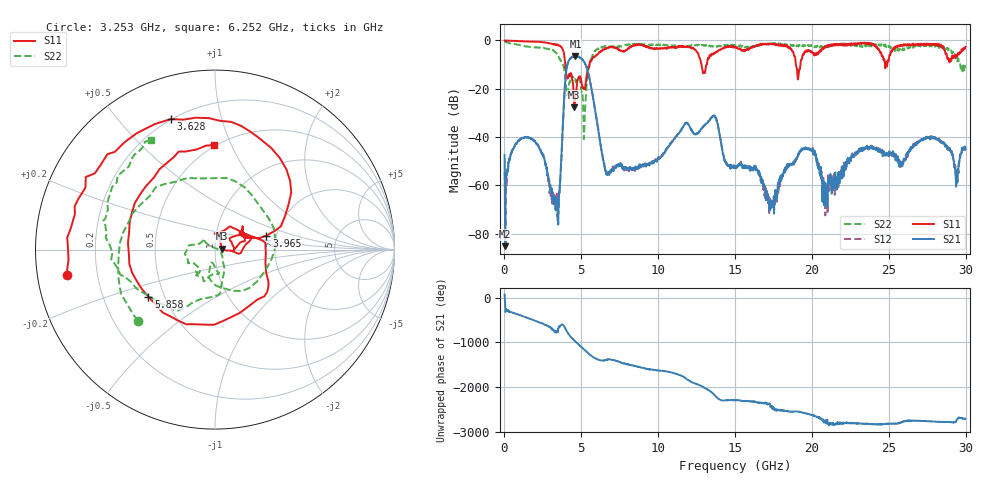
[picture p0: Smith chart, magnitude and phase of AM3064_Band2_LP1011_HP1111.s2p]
# Hz S DB R 50.0
!freq dBS11 angS11 dBS21 angS21 dBS12 angS12 dBS22 angS22
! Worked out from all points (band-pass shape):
!   1600 points, 10 MHz to 29.98 GHz, reference 50 ohm
!   highest |S21| = -6.43 dB at 4.621 GHz (marker M1); lowest = -85.2 dB at 47.49 MHz (marker M2)
!   |S21| within 3 dB of the highest: 4.121 GHz to 5.232 GHz (1.111 GHz wide, 23.8 % of centre)
!   lowest |S11| = -27.7 dB at 4.546 GHz (marker M3), VSWR 1.09, Z = 54.2 + j0.644 ohm
!   |S11| at or under -10 dB: 3.957 GHz to 5.523 GHz (1.566 GHz wide, 33 % of centre); 12.82 GHz to 13.16 GHz (338.7 MHz wide, 2.61 % of centre); 18.95 GHz to 19.25 GHz (298 MHz wide, 1.56 % of centre)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
!   |S22| runs from -40.8 to -0.2 dB; largest |S21 - S12| = 0.01
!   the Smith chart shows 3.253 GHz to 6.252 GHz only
!   S11 on the Smith chart (normalised r, x): 3.253 GHz: 0.09, -0.08; 3.628 GHz: 0.20, +0.70; 3.965 GHz: 1.77, +0.30; 5.858 GHz: 0.41, -0.27; 6.252 GHz: 0.49, +0.87
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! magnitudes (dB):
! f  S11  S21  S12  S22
! 10 MHz  0.0  -47.4  -54.8  -0.2
! 47.49 MHz  -0.1  -85.2  -55.4  -0.4
! 1.659 GHz  -0.5  -40.4  -40.5  -2.7
! 3.253 GHz  -1.6  -64.3  -64.0  -4.6
! 3.628 GHz  -2.3  -57.8  -59.0  -7.9
! 3.965 GHz  -10.5  -15.9  -15.8  -15.9
! 4.546 GHz  -27.7  -6.5  -6.4  -15.9
! 4.621 GHz  -21.2  -6.4  -6.5  -17.0
! 5.015 GHz  -17.6  -7.6  -7.6  -21.5
! 5.858 GHz  -6.8  -27.5  -27.2  -4.9
! 6.252 GHz  -4.7  -43.2  -43.1  -3.0
! 6.739 GHz  -3.2  -54.9  -54.9  -2.4
! 10 GHz  -3.4  -48.5  -48.8  -1.9
! 13.6 GHz  -5.4  -31.4  -31.3  -2.5
! 15 GHz  -2.7  -52.6  -52.0  -1.9
! 17.37 GHz  -1.5  -66.4  -68.3  -1.2
! 19.99 GHz  -4.7  -45.4  -45.7  -2.0
! 20.89 GHz  -2.3  -65.3  -59.9  -2.9
! 25 GHz  -8.1  -48.0  -47.2  -2.2
! 27.86 GHz  -1.6  -40.5  -40.2  -2.1
! 29.4 GHz  -6.3  -57.4  -56.7  -7.0
! 29.98 GHz  -2.7  -45.3  -45.2  -10.3
